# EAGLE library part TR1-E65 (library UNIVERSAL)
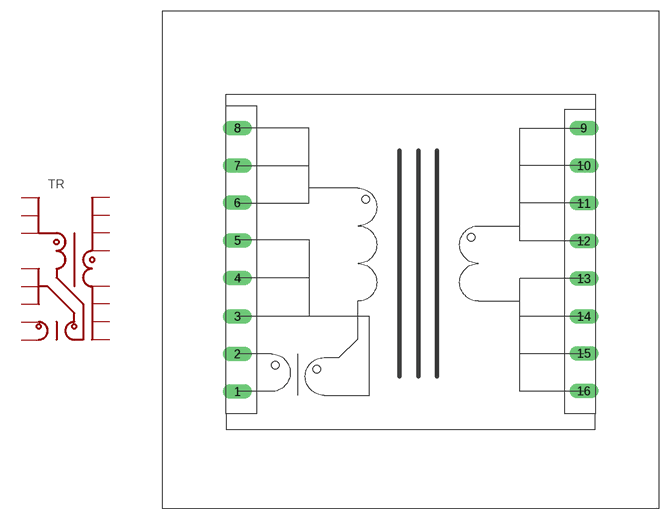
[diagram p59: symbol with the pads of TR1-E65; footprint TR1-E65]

Designator prefix TR

## TR1-E65  [TR1-E65]
1  1
2  2
3  3
4  4
5  5
6  6
7  7
8  8
9  9
10  10
11  11
12  12
13  13
14  14
15  15
16  16

## Footprint TR1-E65 (pad centres in mm)
drill 0.8 pad 1.93 long: 1 10,15.5; 2 10,20.5; 3 10,25.5; 4 10,30.58; 5 10,35.58; 6 10,40.58; 7 10,45.5; 8 10,50.5; 9 56,50.5; 10 56,45.5; 11 56,40.5; 12 56,35.5; 13 56,30.5; 14 56,25.5; 15 56,20.58; 16 56,15.58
